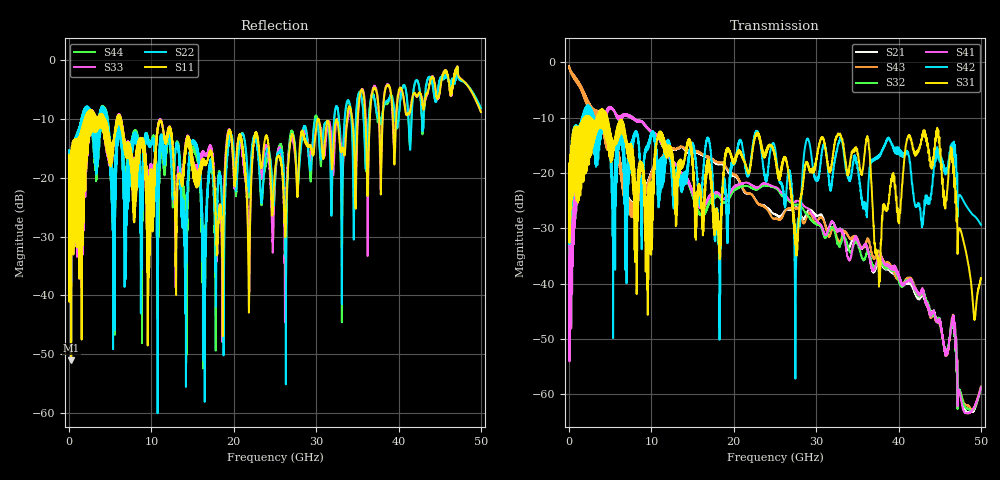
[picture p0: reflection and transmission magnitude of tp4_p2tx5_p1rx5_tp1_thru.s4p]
! 100G CR Analysis
! File: tp4_p2tx5_p1rx5_tp1_thru
! Description: 2m Cu Cable, OSFP, TP1-TP4
! Port Mapping
! Port1 -- P1RX5N
! Port2 -- P2TX5N
! Port3 -- P1RX5P
! Port4 -- P2TX5P
# GHz S MA R 50.00
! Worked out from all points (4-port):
!   5000 points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, 10 MHz to 50 GHz, reference 50 ohm
!   strongest paths, dB at 10 MHz, 12.51 GHz, 25.01 GHz, 37.51 GHz, 50 GHz:
!     S31: -20.5, -17.1, -16.9, -35.9, -39.0
!     S42: -20.6, -20.0, -15.5, -17.2, -29.4
!     S41: -33.3, -18.2, -22.5, -35.5, -58.8
!     S32: -33.3, -18.3, -22.7, -36.2, -58.8
!     S43: -0.7, -15.6, -28.3, -34.4, -58.6
!     S21: -0.7, -15.7, -27.5, -36.5, -58.9
!   lowest |S11| = -51.0 dB at 260 MHz (marker M1), VSWR 1.01, Z = 50.3 + j0.0826 ohm
!   |S11| at or under -10 dB: start of sweep to 1.947 GHz; 6.311 GHz to 30.21 GHz (23.9 GHz wide, 131 % of centre); 30.29 GHz to 33.76 GHz (3.475 GHz wide, 10.9 % of centre)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
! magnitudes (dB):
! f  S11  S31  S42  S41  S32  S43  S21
! 10 MHz  -18.5  -20.5  -20.6  -33.3  -33.3  -0.7  -0.7
! 260 MHz  -51.0  -26.5  -27.8  -48.1  -47.6  -1.7  -1.7
! 5.08 GHz  -16.3  -16.2  -17.9  -8.2  -8.2  -14.3  -14.3
! 36.21 GHz  -22.3  -13.3  -26.4  -33.4  -34.1  -31.8  -33.5
! 37.56 GHz  -7.5  -36.0  -16.9  -35.0  -35.8  -34.0  -36.1
! 44.72 GHz  -6.4  -12.3  -16.6  -46.9  -46.3  -46.9  -47.0
! 50 GHz  -8.8  -39.0  -29.4  -58.8  -58.8  -58.6  -58.9
